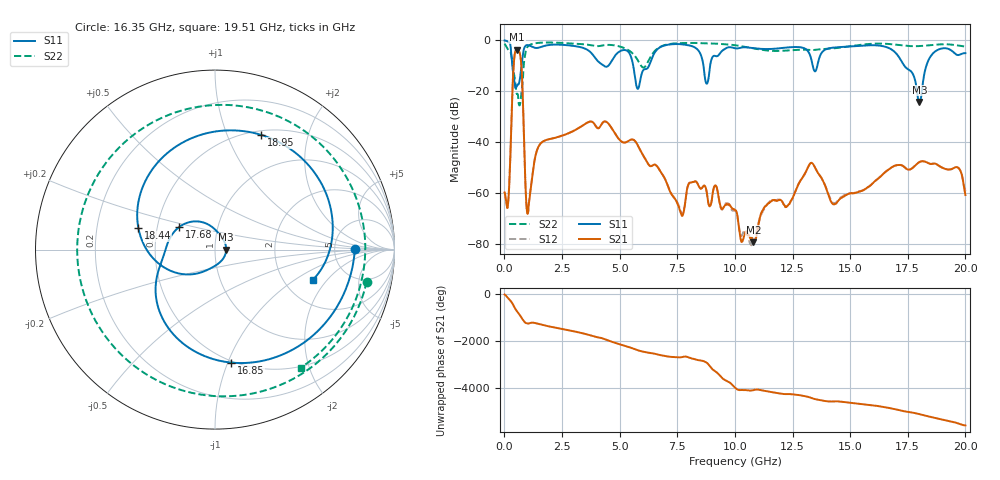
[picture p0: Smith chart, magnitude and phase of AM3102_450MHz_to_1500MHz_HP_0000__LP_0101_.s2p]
!Agilent Technologies,E8364B,MY43040894,A.07.50.67
!Agilent E8364B: A.07.50.67
!Date: Thursday, January 11, 2018 05:15:59
!Correction: S11(Full 2 Port(1,2))
!S21(Full 2 Port(1,2))
!S12(Full 2 Port(1,2))
!S22(Full 2 Port(1,2))
!S2P File: Measurements: S11, S21, S12, S22:
# Hz S  dB  R 50
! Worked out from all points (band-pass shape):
!   1601 points, 10 MHz to 20 GHz, reference 50 ohm
!   highest |S21| = -3.62 dB at 547.2 MHz (marker M1); lowest = -79.2 dB at 10.8 GHz (marker M2)
!   |S21| within 3 dB of the highest: 432.6 MHz to 701.3 MHz (268.7 MHz wide, 47.4 % of centre)
!   lowest |S11| = -24.1 dB at 18 GHz (marker M3), VSWR 1.13, Z = 56.6 + j0.0198 ohm
!   |S11| at or under -10 dB: 346.5 MHz to 745.5 MHz (399 MHz wide, 73.1 % of centre); 5.591 GHz to 6.272 GHz (681.3 MHz wide, 11.5 % of centre); 17.35 GHz to 18.3 GHz (950.8 MHz wide, 5.33 % of centre)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
!   |S22| runs from -25.5 to -0.8 dB; largest |S21 - S12| = 0.0021
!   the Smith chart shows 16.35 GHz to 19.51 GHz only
!   S11 on the Smith chart (normalised r, x): 16.35 GHz: 8.06, +0.04; 16.85 GHz: 0.49, -1.03; 17.68 GHz: 0.65, +0.17; 18.44 GHz: 0.39, +0.12; 18.95 GHz: 0.55, +1.33; 19.51 GHz: 2.84, -1.43
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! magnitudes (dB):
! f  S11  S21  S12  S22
! 10 MHz  0.0  -59.6  -59.4  -1.3
! 172.4 MHz  -0.6  -62.6  -62.7  -3.8
! 547.2 MHz  -17.9  -3.6  -3.6  -21.1
! 722.1 MHz  -11.7  -8.1  -8.1  -22.0
! 1.022 GHz  -1.9  -67.8  -67.7  -2.3
! 1.547 GHz  -2.7  -40.7  -40.7  -0.9
! 3.346 GHz  -2.8  -33.7  -33.7  -1.5
! 5.795 GHz  -19.0  -41.3  -41.3  -7.9
! 6.682 GHz  -3.2  -50.1  -50.0  -3.0
! 10.01 GHz  -3.1  -66.4  -66.6  -1.9
! 10.8 GHz  -3.1  -79.2  -80.2  -3.1
! 13.34 GHz  -8.4  -48.0  -48.0  -3.8
! 14.3 GHz  -2.8  -64.2  -63.8  -3.1
! 16.35 GHz  -2.2  -53.1  -53.0  -1.3
! 16.68 GHz  -3.0  -50.5  -50.5  -1.4
! 16.85 GHz  -3.9  -49.5  -49.5  -1.6
! 17.68 GHz  -12.5  -50.2  -50.2  -2.3
! 18 GHz  -24.1  -47.7  -47.7  -2.2
! 18.44 GHz  -7.1  -48.3  -48.3  -1.9
! 18.95 GHz  -3.2  -49.7  -49.7  -1.6
! 19.51 GHz  -4.9  -50.0  -50.0  -1.8
! 20 GHz  -5.0  -60.6  -59.1  -2.4
